PROGRAM CrcTest

VAR
	aData1		: ARRAY[1..6] OF USINT := [0, 0, 0, 1, 1, 0];
	nCrc1		: BYTE;
	aData2		: ARRAY[1..6] OF USINT := [0, 0, 1, 0, 0, 0];
	nCrc2		: BYTE;
	aData3		: ARRAY[1..6] OF USINT := [1, 0, 0, 0, 0, 1];
	nCrc3		: BYTE;
	
	aData4		: ARRAY[1..6] OF USINT := [16#E, 16#F, 16#F, 16#F, 16#F, 16#E];
	nCrc4		: BYTE;
	aData5		: ARRAY[1..6] OF USINT := [16#F, 16#F, 16#E, 16#F, 16#F, 16#F];
	nCrc5		: BYTE;
	aData6		: ARRAY[1..6] OF USINT := [16#F, 16#F, 16#F, 16#E, 16#E, 16#F];
	nCrc6		: BYTE;
END_VAR

nCrc1 := F_Crc4(aData1);
nCrc2 := F_Crc4(aData2);
nCrc3 := F_Crc4(aData3);
nCrc4 := F_Crc4(aData4);
nCrc5 := F_Crc4(aData5);
nCrc6 := F_Crc4(aData6);

END_PROGRAM
